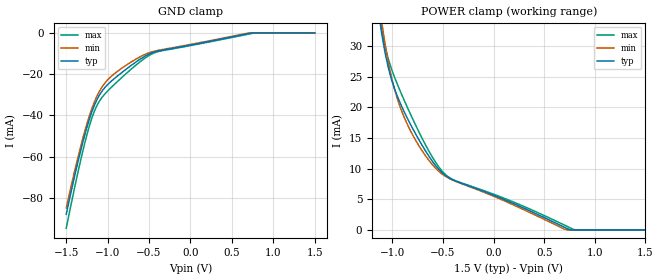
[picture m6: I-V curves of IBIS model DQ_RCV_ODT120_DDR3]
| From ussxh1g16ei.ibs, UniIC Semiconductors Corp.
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|   Model DQ_RCV_ODT120_DDR3
[Model] DQ_RCV_ODT120_DDR3
Model_type Input
Vinl =  0.615V
Vinh =  0.885V
C_comp   1.232pF   1.219pF   1.235pF
[Model Spec]
Vinh   0.885V   0.847V   0.922V
Vinl   0.615V   0.577V   0.652V
[Temperature Range]   25.000   95.000   -40.000
[Voltage Range]   1.500V   1.425V   1.575V
[GND_clamp]
|Voltage   I(typ)   I(min)   I(max)
-1.5V     -87.98mA   -84.92mA   -94.72mA
-1.376V   -65.54mA   -63.2mA    -70.77mA
-1.283V   -50.54mA   -48.68mA   -54.51mA
-1.221V   -41.97mA   -40.31mA   -45.19mA
-1.159V   -35.03mA   -33.38mA   -37.87mA
-1.066V   -28.14mA   -26.1mA    -31.19mA
-973mV    -24.05mA   -21.7mA    -27.1mA
-601mV    -12.59mA   -11.44mA   -13.8mA
-477mV    -9.882mA   -9.319mA   -10.45mA
-384mV    -8.738mA   -8.408mA   -9.006mA
763mV     0A         0A         -95.27uA
1.5V      0A         0A         0A
[POWER_clamp]
|Voltage   I(typ)   I(min)   I(max)
-1.5V     100.7mA    102.3mA    103.6mA
-1.135V   35.28mA    37.51mA    35.73mA
-1.104V   31.83mA    33.71mA    32.48mA
-1.073V   28.93mA    30.36mA    29.94mA
-1.011V   24.65mA    25.04mA    26.34mA
-949mV    21.71mA    21.27mA    23.66mA
-887mV    19.38mA    18.5mA     21.27mA
-701mV    13.65mA    12.77mA    14.76mA
-484mV    8.973mA    8.826mA    9.158mA
725mV     235.4uA    0A         596uA
818mV     0A         0A         0A
1.5V      0A         0A         0A
